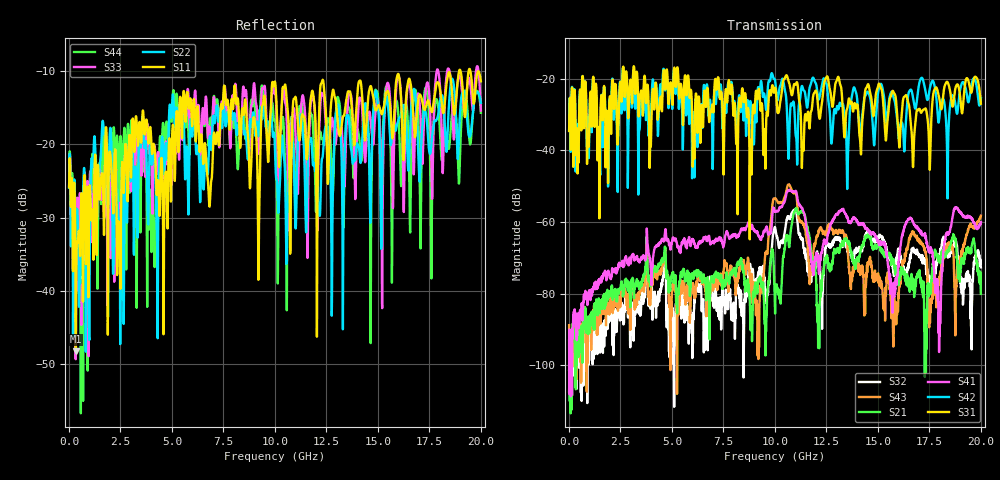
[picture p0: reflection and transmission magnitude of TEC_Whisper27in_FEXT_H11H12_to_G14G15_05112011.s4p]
! Tyco Electronics
! H11H12-G14G15_FEXT
!! PART DESCRIPTION: Whisper 27in Megtron 6 VLP-HVLP-VLP Channel Model, bulkhead 2.4mm test pts
!! MODEL DESCRIPTION: System 4-port S-parameter
!! MODEL STATUS: Measured
!! MODEL GEOMETRY: Channel Model
!! MODEL FREQUENCY RANGE: DC to 20.000 GHz in 10.000 MHz frequency steps
!! MODEL EDGE RATE LIMITATION: 25.00 ps (Using conservative 0.5/Fmax rule of thumb)
!! TIME-DOMAIN TRANSFORM CAUTIONS:
!! 1.) Do not simulate transient edge rates faster than the number listed above.  Edge rates faster than this number
!!  contain significant spectral content at frequencies above the model's highest frequency.
!! 2.) Even when simulating edge rates that are slower than the number listed above, be aware that the best time
!!  resolution possible with a direct iFFT is (1 / 2Fmax).  As a result, time resolution is typically not adequate
!!  for most time-domain simulations unless tricks such as windowing are used to minimize leakage and aliasing.
!! 3.) Because the model has a uniform frequency step, a direct iFFT will result in an impulse that that has a time
!!  length given by either (1 / Fstep) or (1 / 2Fstep), depending on the transform being used.  Care has been taken
!!  in selecting the frequency step to ensure a settled impulse response for the model.  Therefore, convolution with
!!  the model's impulse response should present no issues.  However, if directly concatenating s-parameter models
!!  in the frequency domain a user must either interpolate necessary interim frequencies or complete impulse response
!!  zero-padding.  Impulse response zero-padding is more difficult, but more accurate.
!! PORT DEFINITIONS:
!! Port  1  ----->  Side A  H11  G14  Side B  <-----  Port  2
!! Port  3  ----->  Side A  H12  G15  Side B  <-----  Port  4
! Point-to-Point link (differential)  !
! Connectors:  !
!  1: STRADA Whisper  !
! Materials:  !
!  Backplane: Megtron-6 HVLP  !
!  Daughtercard: Megtron-6 VLP  !
! Stack-up:  !
!  Backplane: 20 layers, 200mil thick  !
!  Daughtercard: 14 layers, 110mil thick  !
! Trace Length:  !
!  Backplane: 17in  !
!  Daightercards: 5in  !
! Trace Width:  !
!  Backplane: 8-13-8 mils  !
!  Daughtercards: 6-9-6 mils  !
! Geometry:  !
!  Backplane: Stripline  !
!  Daughtercards: Stripline  !
! Freq. Range: 0 GHz - 20 GHz  !
! Note1: non-mixed-mode s-parameters  !
! Note2: channel includes 2.4mm test points  !
! Created Wed May 11 14:44:14 2011
! 4 Port Network Data from SP1.SP block
! freq  magS11  angS11  magS12  angS12  magS13  angS13  magS14  angS14
!  magS21  angS21  magS22  angS22  magS23  angS23  magS24  angS24
!  magS31  angS31  magS32  angS32  magS33  angS33  magS34  angS34
!  magS41  angS41  magS42  angS42  magS43  angS43  magS44  angS44
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# hz S ma R 50
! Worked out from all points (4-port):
!   2000 points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, 10 MHz to 20 GHz, reference 50 ohm
!   strongest paths, dB at 10 MHz, 5.01 GHz, 10.01 GHz, 15.01 GHz, 20 GHz:
!     S31: -34.6, -26.0, -22.5, -22.0, -27.0
!     S42: -34.4, -28.1, -20.5, -23.8, -25.4
!     S41: -93.1, -65.5, -57.0, -65.0, -60.0
!     S21: -101.5, -75.1, -85.6, -66.2, -80.1
!     S43: -88.8, -79.1, -53.4, -74.3, -58.2
!     S32: -107.5, -85.3, -61.6, -64.7, -72.7
!   lowest |S11| = -48.3 dB at 340 MHz (marker M1), VSWR 1.01, Z = 50.2 + j0.338 ohm
!   |S11| at or under -10 dB: start of sweep to 18.94 GHz; 19.01 GHz to 19.4 GHz (387.8 MHz wide, 2.02 % of centre); 19.49 GHz to 19.86 GHz (368.8 MHz wide, 1.87 % of centre)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
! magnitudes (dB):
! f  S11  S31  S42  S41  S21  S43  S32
! 10 MHz  -25.9  -34.6  -34.4  -93.1  -101.5  -88.8  -107.5
! 340 MHz  -48.3  -41.4  -42.0  -89.7  -106.7  -100.3  -100.0
! 9.16 GHz  -25.2  -25.6  -23.4  -63.3  -77.8  -97.4  -75.5
! 11.01 GHz  -13.5  -21.6  -35.9  -51.3  -56.2  -51.9  -56.8
! 12.13 GHz  -17.6  -30.0  -25.8  -73.8  -89.2  -62.3  -69.5
! 15.75 GHz  -18.3  -23.6  -25.0  -80.3  -71.7  -94.8  -72.9
! 20 GHz  -11.4  -27.0  -25.4  -60.0  -80.1  -58.2  -72.7
